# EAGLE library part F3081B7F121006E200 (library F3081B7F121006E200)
FFC & FPC Connectors F308-1B7F1-21006-E20 #VALUE! Source: Datasheet
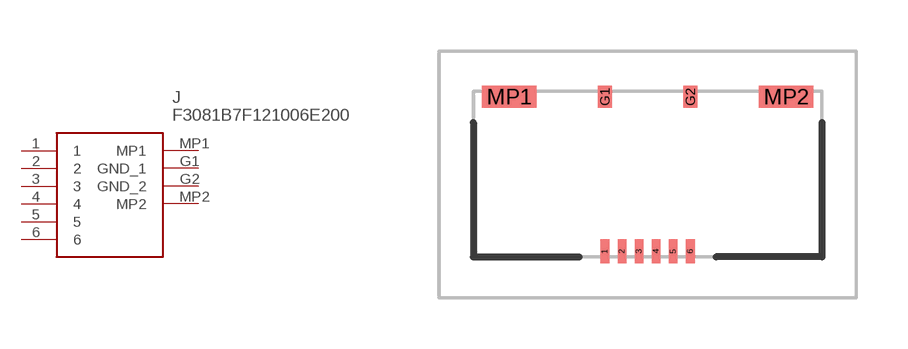
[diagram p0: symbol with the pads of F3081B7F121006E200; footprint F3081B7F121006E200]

Designator prefix J

## F3081B7F121006E200 (Description: FFC & FPC Connectors F308-1B7F1-21006-E20 #VALUE!; Height: 2.8mm; Manufacturer_Name: Amphenol; Manufacturer_Part_Number: F3081B7F121006E200; Mouser_Part_Number: 649-F3081B7F006E200; Mouser_Price-Stock: https://www.mouser.co.uk/ProductDetail/Amphenol-FCI/F3081B7F121006E200?qs=OlC7AqGiEDlbHOY63ODzcg%3D%3D)  [F3081B7F121006E200]
1  1
2  2
3  3
4  4
5  5
6  6
G1  GND_1
G2  GND_2
MP1  MP1
MP2  MP2

## Footprint F3081B7F121006E200 (pad centres in mm)
F3081B7F121006E200-4
smd 0.25 x 0.7: 1 -1.25,-2.263; 2 -0.75,-2.263; 3 -0.25,-2.263; 4 0.25,-2.263; 5 0.75,-2.263; 6 1.25,-2.263
smd 0.4 x 0.65: G1 -1.25,2.262; G2 1.25,2.262
smd 1.6 x 0.65: MP1 -4.05,2.262; MP2 4.05,2.262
